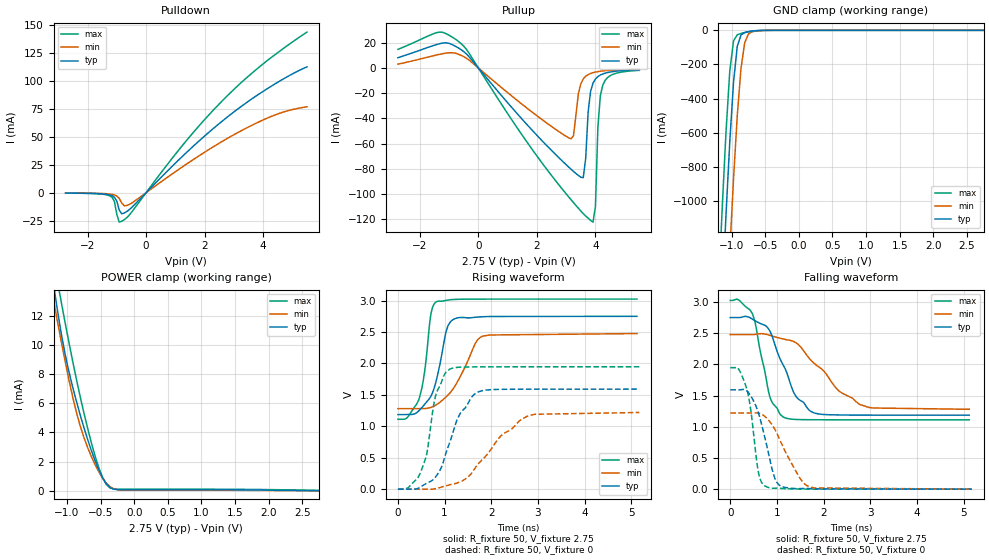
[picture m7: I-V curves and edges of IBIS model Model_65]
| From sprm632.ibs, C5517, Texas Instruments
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| Model based on original model for BC3340CTSCHYPD
|   Sub model SR0_VSS_SR1_VSS_PD_ON_IND_2P75
[model]   Model_65
|[Description]  [2.75V-I/O-PD-X, IND]
|   PD,IND,
|[Input Load]   PD
|[Output Drive]
|Voltage   2.75V
|Mode   I/O
Model_type   I/O
Polarity   Non-Inverting
Enable   Active-Low
Vinl =  0.7
Vinh =  1.7
Cref =  15.0000pF
Rref =  100.0000M
Vref =  0V
Vmeas =  1.375
C_comp   2.1456989p   2.0494201p   2.2784851p
[Model Spec]
Vinl   0.7   0.7   0.7
Vinh   1.7   1.7   1.7
[Temperature Range]   25   105   -40
[Voltage Range]   2.75   2.475   3.025
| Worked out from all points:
|   slope of the pulldown table from 0 to 0.412 V, typ, clamps not added: 37.1 ohm
|   slope of the pullup table from 0 to 0.412 V, typ, clamps not added: 35.9 ohm
|   GND clamp passes 1 mA (typ) near -0.57 V on its own axis
|   POWER clamp passes 1 mA (typ) near -0.48 V on its own axis
|   rising waveform, R_fixture 50, V_fixture 2.75: 20-80 % time 291ps typ, 507ps min, 205ps max; typ from 1.19 V to 2.75 V
|   rising waveform, R_fixture 50, V_fixture 0: 20-80 % time 502ps typ, 894ps min, 294ps max; typ from 0 V to 1.59 V
|   falling waveform, R_fixture 50, V_fixture 2.75: 20-80 % time 495ps typ, 894ps min, 303ps max; typ from 2.75 V to 1.19 V
|   falling waveform, R_fixture 50, V_fixture 0: 20-80 % time 316ps typ, 497ps min, 207ps max; typ from 1.59 V to 0 V
[POWER_clamp]
-2.75V    68.54mA    53.4mA     82.8mA
-1.25V    15.8mA     14.35mA    17.53mA
-1.194V   14.01mA    12.94mA    15.84mA
-1.139V   12.31mA    11.56mA    14.33mA
-1.083V   10.75mA    10.21mA    12.92mA
-972.2mV  8.203mA    7.648mA    10.22mA
-805.6mV  5.244mA    4.485mA    6.506mA
-638.9mV  2.782mA    2.364mA    3.323mA
-527.8mV  1.441mA    1.31mA     1.596mA
-361.1mV  223.7uA    277.8uA    199.5uA
-138.9mV  61.83uA    37.73uA    104.2uA
2.75V     -8.84nA    -15.87uA   24.28uA
[Pulldown]
-2.75V    -308.5uA   -227.6uA   -349uA
-1.25V    -1.93mA    -1.163mA   -2.672mA
-1.083V   -4.054mA   -1.991mA   -7.636mA
-1V       -7.547mA   -2.954mA   -19.38mA
-916.7mV  -15.6mA    -5.046mA   -26.43mA
-833.3mV  -18.95mA   -9.139mA   -25.59mA
-750mV    -18.23mA   -11.68mA   -24.25mA
-500mV    -13.48mA   -9.45mA    -17.63mA
1.333V    34.87mA    24.79mA    45.26mA
2.5V      61.98mA    44.41mA    79.58mA
4.25V     95.04mA    68.08mA    120.7mA
5.5V      112.9mA    77.06mA    144mA
[Pullup]
-2.75V    8.15mA     3.088mA    14.75mA
-1.333V   19.2mA     10.81mA    28.46mA
-583.3mV  14.38mA    9.918mA    19.15mA
3.167V    -80.24mA   -56.1mA    -104.4mA
3.583V    -86.93mA   -8.662mA   -115.4mA
3.667V    -71.56mA   -6.559mA   -117.3mA
3.75V     -34.81mA   -5.246mA   -119mA
3.917V    -11.98mA   -3.72mA    -122.2mA
4V        -8.725mA   -3.242mA   -109.7mA
4.083V    -6.819mA   -2.87mA    -47.03mA
4.25V     -4.711mA   -2.331mA   -13.63mA
5.5V      -1.388mA   -959.6uA   -1.855mA
[GND_clamp]
-2.75V    -17.03A    -17.67A    -16.58A
-1.194V   -2.025A    -2.722A    -1.509A
-1.139V   -1.54A     -2.231A    -1.032A
-1.083V   -1.078A    -1.755A    -593.8mA
-1.028V   -655mA     -1.299A    -239.9mA
-972.2mV  -306mA     -874.1mA   -62.06mA
-916.7mV  -94.94mA   -503mA     -26.47mA
-861.1mV  -27.25mA   -223.2mA   -18.07mA
-805.6mV  -13.1mA    -72.24mA   -12.46mA
-750mV    -8.089mA   -21.21mA   -7.808mA
-694.4mV  -4.87mA    -8.039mA   -4.202mA
2.75V     61.47uA    87.87uA    104.1uA
[Ramp]
dV/dt_f  0.9501825/0.49755523n 0.72669005/0.89856808n  1.1604743/0.30652674n
dV/dt_r 0.95689585/0.50305895n 0.73349807/0.90020925n  1.1699958/0.29455498n
R_load = 50
[Rising Waveform]
R_fixture = 50
V_fixture = 2.75
V_fixture_min = 2.475
V_fixture_max = 3.025
0s        1.186V     1.28V      1.111V
186.5ps   1.187V     1.28V      1.129V
448ps     1.246V     1.281V     1.428V
573.5ps   1.351V     1.282V     1.878V
703.4ps   1.475V     1.299V     2.769V
819.3ps   1.722V     1.341V     2.978V
1.069ns   2.594V     1.494V     3.007V
1.257ns   2.72V      1.685V     3.019V
1.811ns   2.742V     2.432V     3.022V
5.12ns    2.749V     2.474V     3.023V
[Rising Waveform]
R_fixture = 50
V_fixture = 0
V_fixture_min = 0
V_fixture_max = 0
0s        0V         0V         0V
475.8ps   32.19mV    0V         252.7mV
621.5ps   95.97mV    0V         573.5mV
809.2ps   197.1mV    8.658mV    1.493V
1.104ns   732.3mV    68.68mV    1.906V
1.347ns   1.221V     119.6mV    1.94V
1.795ns   1.564V     461.1mV    1.945V
2.212ns   1.588V     851.3mV    1.946V
2.836ns   1.59V      1.175V     1.946V
5.172ns   1.591V     1.219V     1.946V
[Falling Waveform]
R_fixture = 50
V_fixture = 2.75
V_fixture_min = 2.475
V_fixture_max = 3.025
0s        2.748V     2.475V     3.023V
202.3ps   2.748V     2.475V     3.019V
471.6ps   2.724V     2.475V     2.814V
841.9ps   2.54V      2.465V     1.496V
1.135ns   1.986V     2.405V     1.155V
1.413ns   1.481V     2.343V     1.116V
1.818ns   1.216V     2.002V     1.112V
2.338ns   1.189V     1.568V     1.111V
2.965ns   1.186V     1.31V      1.111V
5.12ns    1.185V     1.28V      1.111V
[Falling Waveform]
R_fixture = 50
V_fixture = 0
V_fixture_min = 0
V_fixture_max = 0
0s        1.591V     1.22V      1.946V
184.3ps   1.591V     1.22V      1.918V
355.9ps   1.574V     1.22V      1.6V
443.7ps   1.487V     1.22V      1.243V
602.7ps   1.224V     1.218V     271.7mV
761.6ps   762.1mV    1.151V     43.88mV
898.6ps   311.4mV    1.028V     14.86mV
1.035ns   75.43mV    836.2mV    16.71mV
1.693ns   9.106mV    39.48mV    1.364mV
5.172ns   11.9uV     112.5uV    0V
